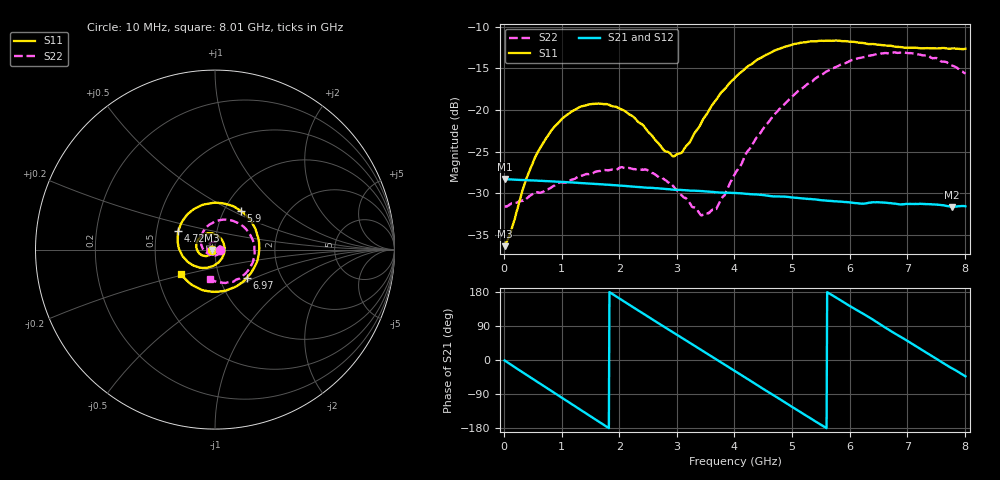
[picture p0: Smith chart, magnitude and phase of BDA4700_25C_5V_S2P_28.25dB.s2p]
!Agilent Technologies,E5071B,MY42404982,A.09.10
!Date: Mon Oct 20 13:40:47 2025
!Data & Calibration Information:
!Freq	S11:SOLT2(ON)	S21:SOLT2(ON)	S12:SOLT2(ON)	S22:SOLT2(ON)
# Hz S RI R 50
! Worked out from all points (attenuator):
!   801 points, 10 MHz to 8.01 GHz, reference 50 ohm
!   highest |S21| = -28.31 dB at 10 MHz (marker M1); lowest = -31.7 dB at 7.77 GHz (marker M2)
!   lowest |S11| = -36.4 dB at 10 MHz (marker M3), VSWR 1.03, Z = 48.5 - j0.128 ohm
!   |S11| at or under -10 dB: start of sweep to end of sweep
!   |S22| runs from -32.7 to -13.0 dB; largest |S21 - S12| = 0.00033
!   S11 on the Smith chart (normalised r, x): 10 MHz: 0.97, -0.00; 4.72 GHz: 0.65, +0.14; 5.9 GHz: 1.19, +0.55; 6.97 GHz: 1.35, -0.45; 8.01 GHz: 0.66, -0.19
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1e7  -0.0151 -0.00132  0.0384 -0.000823  0.0384 -0.000867  0.0262 -0.000809
1.2e8  -0.0162 -0.00906  0.0373 -0.00813  0.0372 -0.00815  0.0266 -0.0058
3.8e8  -0.0268 -0.0268  0.0297 -0.0234  0.0297 -0.0235  0.0214 -0.0197
5.9e8  -0.0435 -0.0357  0.0193 -0.0321  0.0193 -0.0322  0.0134 -0.029
9.9e8  -0.0837 -0.0242  -0.00549 -0.0365  -0.00551 -0.0365  -0.014 -0.0338
1.35e9  -0.1043 0.0147  -0.0252 -0.0261  -0.0252 -0.0262  -0.036 -0.0179
2.06e9  -0.0432 0.0903  -0.0322 0.0137  -0.0322 0.0138  -0.0311 0.0326
2.68e9  0.0439 0.0451  -0.00423 0.0335  -0.00422 0.0335  0.0127 0.0375
2.93e9  0.0527 0.000466  0.00949 0.0318  0.00955 0.0318  0.0247 0.0248
3.06e9  0.0492 -0.0244  0.016 0.0289  0.0159 0.0289  0.0274 0.0149
3.44e9  -0.000482 -0.0858  0.0295 0.0137  0.0295 0.0137  0.0187 -0.0139
3.69e9  -0.0556 -0.1017  0.0319 0.000682  0.032 0.000601  0.000651 -0.0255
4.01e9  -0.1337 -0.0808  0.0276 -0.0155  0.0276 -0.0154  -0.0322 -0.0257
4.72e9  -0.204 0.1053  -0.00359 -0.0299  -0.00355 -0.03  -0.0797 0.054
5.35e9  -0.0559 0.2526  -0.0267 -0.0115  -0.0266 -0.0116  -0.0152 0.1476
5.9e9  0.1425 0.2169  -0.0247 0.0131  -0.0247 0.0131  0.1068 0.1573
6.26e9  0.2272 0.1094  -0.0136 0.0237  -0.0134 0.0238  0.1808 0.1039
6.68e9  0.2375 -0.0557  0.00485 0.0271  0.00496 0.0272  0.22 0.000533
6.97e9  0.1791 -0.1556  0.0161 0.0219  0.0161 0.0218  0.2071 -0.077
7.37e9  0.0384 -0.2323  0.026 0.00744  0.0261 0.00741  0.1374 -0.1615
7.77e9  -0.1216 -0.2006  0.0243 -0.00945  0.0243 -0.00951  0.0289 -0.1832
8.01e9  -0.1899 -0.1358  0.0192 -0.018  0.0194 -0.0181  -0.0302 -0.1624
